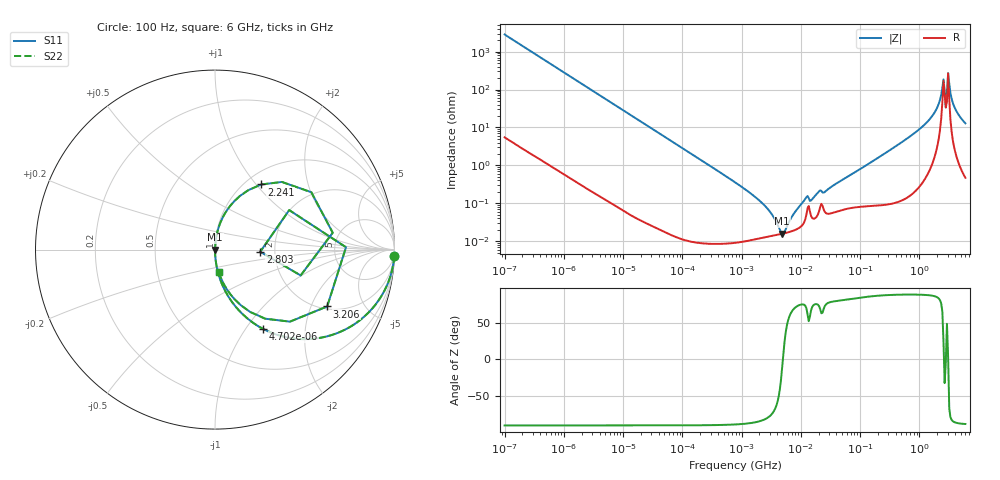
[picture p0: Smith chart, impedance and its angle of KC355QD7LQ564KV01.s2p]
!Murata Part Number: KC355QD7LQ564KV01
!These Parameters are Measured in Series Mode Connection
!Data Generated on Jun 19, 2026
!  o--ll--o
!Port1  Port2
!  o------o
!Operation Temp=25[degC], DC Bias Voltage=0[V]
!Freq. Start=100[Hz] Stop=6[GHz] 401[Steps]
# Hz S RI R 50
!Freq.(Hz) S11(Real) S11(Imag) S21(Real) S21(Imag) S12(Real) S12(Imag) S22(Real) S22(Imag)
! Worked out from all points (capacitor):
!   401 points, 100 Hz to 6 GHz, reference 50 ohm
!   read as one part in series: C = 561 nF near 109 Hz
!   lowest |Z| = 15.9 mohm at 4.857 MHz (marker M1)
!   series resonance near 4.978 MHz, so ESL is about 1.8 nH
!   S11 on the Smith chart (normalised r, x): 100 Hz: 1, -57; 4.702 kHz: 1.00, -1.21; 2.241 GHz: 1.18, +1.07; 2.803 GHz: 1.67, -0.04; 3.206 GHz: 2.11, -2.63; 6 GHz: 1.01, -0.26
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100  0.9987 -0.0352  0.00131 0.0352  0.00131 0.0352  0.9987 -0.0352
717  0.9397 -0.237  0.0603 0.237  0.0603 0.237  0.9397 -0.237
2008  0.6673 -0.4701  0.3327 0.4701  0.3327 0.4701  0.6673 -0.4701
4702  0.269 -0.4424  0.731 0.4424  0.731 0.4424  0.269 -0.4424
11009  0.0634 -0.2425  0.9366 0.2425  0.9366 0.2425  0.0634 -0.2425
40335  0.0052 -0.0705  0.9948 0.0705  0.9948 0.0705  0.0052 -0.0705
774597  0.000103 -0.00358  0.9999 0.00358  0.9999 0.00358  0.000103 -0.00358
2481164  0.000128 -0.000847  0.9999 0.000847  0.9999 0.000847  0.000128 -0.000847
4856642  0.000157 -2.73e-05  0.9998 2.73e-05  0.9998 2.73e-05  0.000157 -2.73e-05
1.189169e7  0.000378 0.00125  0.9996 -0.00125  0.9996 -0.00125  0.000378 0.00125
1.555665e7  0.000411 0.00122  0.9996 -0.00122  0.9996 -0.00122  0.000411 0.00122
2.035112e7  0.000623 0.00197  0.9994 -0.00197  0.9994 -0.00197  0.000623 0.00197
3.124326e8  0.00156 0.0247  0.9984 -0.0247  0.9984 -0.0247  0.00156 0.0247
1.565993e9  0.0391 0.1709  0.9609 -0.1709  0.9609 -0.1709  0.0391 0.1709
1.95892e9  0.1066 0.2689  0.8934 -0.2689  0.8934 -0.2689  0.1066 0.2689
2.240541e9  0.2586 0.363  0.7414 -0.363  0.7414 -0.363  0.2586 0.363
2.450438e9  0.5368 0.3196  0.4632 -0.3196  0.4632 -0.3196  0.5368 0.3196
2.802721e9  0.2518 -0.0121  0.7482 0.0121  0.7482 0.0121  0.2518 -0.0121
3.205649e9  0.6249 -0.3167  0.3751 0.3167  0.3751 0.3167  0.6249 -0.3167
3.505958e9  0.2795 -0.385  0.7205 0.385  0.7205 0.385  0.2795 -0.385
4.009986e9  0.1091 -0.2767  0.8909 0.2767  0.8909 0.2767  0.1091 -0.2767
6e9  0.0207 -0.1251  0.9793 0.1251  0.9793 0.1251  0.0207 -0.1251
